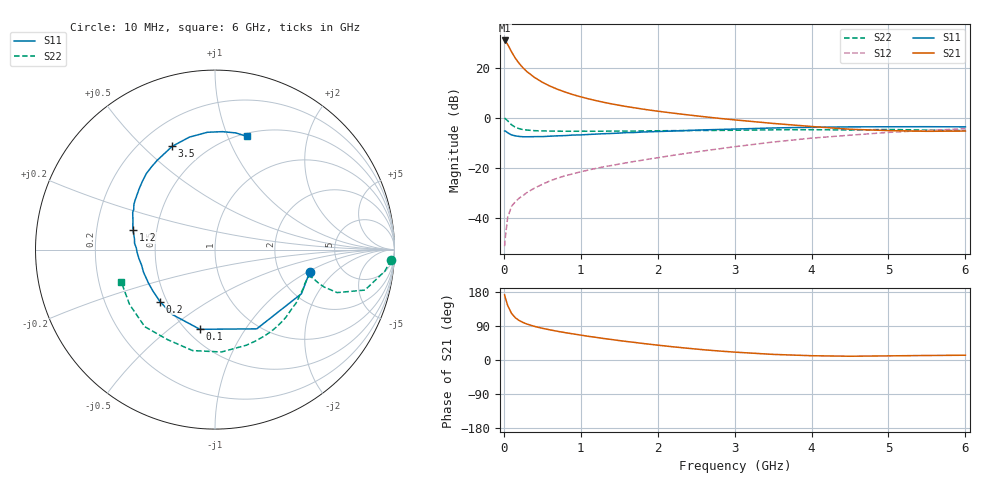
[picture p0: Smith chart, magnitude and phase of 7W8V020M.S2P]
! Infineon Technologies  Discrete & RF Semiconductors
! BFS17W
! Si NPN RF Bipolar Junction Transistor in SOT323
! VCE = 8 V  IC = 20 mA
! Common Emitter S-Parameters:  August  1999
# GHz  S  MA  R  50
!  f  S11  S21  S12  S22
! GHz  MAG  ANG  MAG  ANG  MAG  ANG  MAG  ANG
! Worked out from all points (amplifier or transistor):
!   36 points, 10 MHz to 6 GHz, reference 50 ohm
!   highest |S21| = 30.9 dB at 10 MHz (marker M1)
!   |S21| within 3 dB of that: start of sweep to 73.7 MHz
!   unconditionally stable (mu >= 1): 312.6 MHz to 2.042 GHz; 5.57 GHz to end of sweep
!   at 250 MHz: K = 0.95, MSG = 25.5 dB, |S12| = -31.2 dB
!   at 1.4 GHz: K = 1.14, MAG = 10.0 dB, |S12| = -19.1 dB
!   at 6 GHz: K = 1.03, MAG = -1.5 dB, |S12| = -4.4 dB
!   S11 on the Smith chart (normalised r, x): 10 MHz: 2.94, -1.06; 100 MHz: 0.58, -0.65; 200 MHz: 0.46, -0.32; 1.2 GHz: 0.37, +0.10; 3.5 GHz: 0.33, +0.62; 6 GHz: 0.53, +1.17
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0.01  0.5419 -13.6  34.98 171.8  0.0027 79.0  0.9828 -3.3
0.02  0.5408 -27.0  34.02 163.8  0.0041 85.2  0.9542 -7.2
0.05  0.4991 -62.2  29.09 143.8  0.0102 67.9  0.8655 -15.1
0.1  0.4519 -100.7  20.71 123.1  0.0169 60.6  0.7213 -19.4
0.15  0.433 -123.4  15.39 111.3  0.0209 60.0  0.6414 -18.9
0.2  0.4216 -136.6  12.1 104.1  0.0247 62.9  0.6025 -17.8
0.25  0.4158 -146.1  9.887 98.9  0.0277 62.8  0.5779 -16.7
0.3  0.415 -152.8  8.347 94.9  0.0319 64.7  0.5659 -16.2
0.4  0.4177 -162.3  6.352 88.6  0.0392 66.6  0.5496 -15.8
0.5  0.4184 -168.4  5.119 83.7  0.0466 68.5  0.544 -16.2
0.6  0.4268 -173.3  4.274 79.5  0.0545 69.7  0.54 -17.1
0.7  0.4337 -177.6  3.688 75.7  0.0619 70.2  0.538 -18.3
0.9  0.4497 175.5  2.886 68.9  0.0756 71.3  0.5353 -21.4
1.1  0.4617 169.0  2.381 62.4  0.0898 72.0  0.5367 -25.2
1.2  0.4697 166.6  2.19 59.7  0.097 72.5  0.5364 -27.2
1.6  0.5031 155.7  1.663 48.7  0.1259 73.6  0.5398 -35.9
2.2  0.5411 141.4  1.233 34.8  0.1768 74.9  0.5503 -50.7
2.8  0.5811 127.5  0.97 23.7  0.2388 73.2  0.5573 -66.8
3.5  0.6229 112.5  0.768 14.8  0.3259 68.3  0.5715 -86.4
4.5  0.6551 93.7  0.587 9.9  0.4468 56.0  0.5669 -117.8
5.5  0.6604 79.8  0.534 11.9  0.5565 42.8  0.5656 -147.4
6  0.6552 74.4  0.54 12.6  0.6 36.2  0.5525 -160.8
